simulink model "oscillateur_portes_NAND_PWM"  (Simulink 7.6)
settings: Solver=ode23tb  StartTime=0.0  StopTime=0.01  RelTol=1e-3
InitFcn:
  | clc
StopFcn:
  | close all
  | load es.mat
  | plot(es(1,:),es(2,:))
  | title('Oscillateur PWM à portes NAND')
  | xlabel('temps')
  | grid
  | 
  | delete *.mat
libraries: fl_lib x6, elec_lib x3, nesl_utility x2

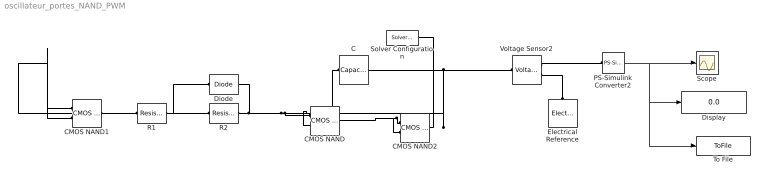
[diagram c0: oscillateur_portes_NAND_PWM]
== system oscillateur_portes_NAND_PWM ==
  C : fl_lib/Electrical/Electrical Elements/Capacitor  DialogController=NetworkEngine.DynNeDlgSource  SystemSampleTime=-1  c=1e-6 F  v0=5 V  r=1e-6 Ohm  g=0 1/Ohm  i_Log=off  v_Log=off  vc_Log=off  LocalVarNames=|i|v|vc  LocalVarDescs=|i|v|Internal variable for voltage across capacitor term  LocalVarLogging=[0 0 0]
  CMOS NAND : elec_lib/Integrated Circuits/Logic/CMOS NAND  DialogController=NetworkEngine.DynNeDlgSource  SystemSampleTime=-1  V_IL=2 V  V_IH=3 V  C_IN=5 pF  output_type=1  V_OL=0 V  V_OH=5 V  V_CC=5 V  V_meas=5 V  R_OUT=25 Ohm  R_OH=[ 25 250 ] Ohm  I_OH=63 mA  R_OL=[ 30 800 ] Ohm  I_OL=-45 mA  Delay=25 ns  Ron=5 Ohm  Vf=0.6 V  output_state=1  LocalVarLogging=[]
  CMOS NAND1 : elec_lib/Integrated Circuits/Logic/CMOS NAND  DialogController=NetworkEngine.DynNeDlgSource  SystemSampleTime=-1  V_IL=2 V  V_IH=3 V  C_IN=5 pF  output_type=1  V_OL=0 V  V_OH=5 V  V_CC=5 V  V_meas=5 V  R_OUT=25 Ohm  R_OH=[ 25 250 ] Ohm  I_OH=63 mA  R_OL=[ 30 800 ] Ohm  I_OL=-45 mA  Delay=25 ns  Ron=5 Ohm  Vf=0.6 V  output_state=1  LocalVarLogging=[]
  CMOS NAND2 : elec_lib/Integrated Circuits/Logic/CMOS NAND  DialogController=NetworkEngine.DynNeDlgSource  SystemSampleTime=-1  V_IL=2 V  V_IH=3 V  C_IN=5 pF  output_type=1  V_OL=0 V  V_OH=5 V  V_CC=5 V  V_meas=5 V  R_OUT=25 Ohm  R_OH=[ 25 250 ] Ohm  I_OH=63 mA  R_OL=[ 30 800 ] Ohm  I_OL=-45 mA  Delay=25 ns  Ron=5 Ohm  Vf=0.6 V  output_state=1  LocalVarLogging=[]
  Diode : fl_lib/Electrical/Electrical Elements/Diode  DialogController=NetworkEngine.DynNeDlgSource  SystemSampleTime=-1  Vf=0.6 V  Ron=0.3 Ohm  Goff=1e-8 1/Ohm  i_Log=off  v_Log=off  LocalVarNames=|i|v  LocalVarDescs=|i|v  LocalVarLogging=[0 0]
  Display : Display
  Electrical Reference : fl_lib/Electrical/Electrical Elements/Electrical Reference  DialogController=NetworkEngine.DynNeDlgSource  SystemSampleTime=-1  i_Log=off  LocalVarNames=|i  LocalVarDescs=|i  LocalVarLogging=0
  PS-Simulink Converter2 : nesl_utility/PS-Simulink Converter  DialogController=NetworkEngine.DynNeUtilDlgSource  SystemSampleTime=-1  PhysicalDomain=network_engine_domain  LeftPortType=input  RightPortType=output  SubClassName=ps_output  Unit=1  AffineConversion=off
  R1 : fl_lib/Electrical/Electrical Elements/Resistor  DialogController=NetworkEngine.DynNeDlgSource  SystemSampleTime=-1  R=0.47 kOhm  i_Log=off  v_Log=off  LocalVarNames=|i|v  LocalVarDescs=|i|v  LocalVarLogging=[0 0]
  R2 : fl_lib/Electrical/Electrical Elements/Resistor  DialogController=NetworkEngine.DynNeDlgSource  SystemSampleTime=-1  R=1.2 kOhm  i_Log=off  v_Log=off  LocalVarNames=|i|v  LocalVarDescs=|i|v  LocalVarLogging=[0 0]
  Scope : Scope
  Solver Configuration : nesl_utility/Solver Configuration  DialogController=NetworkEngine.DynNeUtilDlgSource  SystemSampleTime=-1  PhysicalDomain=network_engine_domain  LeftPortType=input  RightPortType=generic  SubClassName=solver  Accelerate=off  Profile=off  ResidualTolerance=1e-9  MaxNonlinIter=12  MaxModeIter=2  DoFixedCost=off  UseLocalSampling=off  DoDC=off  LinearAlgebra=Sparse  LocalSolverSampleTime=.001  LocalSolverChoice=NE_BACKWARD_EULER_ADVANCER  UseLocalSolver=off
  To File : ToFile  Filename=es.mat  MatrixName=es
  Voltage Sensor2 : fl_lib/Electrical/Electrical Sensors/Voltage Sensor  DialogController=NetworkEngine.DynNeDlgSource  SystemSampleTime=-1  i1_Log=off  v1_Log=off  LocalVarNames=|i1|v1  LocalVarDescs=|i1|v1  LocalVarLogging=[]
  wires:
  PS-Simulink Converter2/1 -> Scope/1, Display/1, To File/1
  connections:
  R2/RConn1 -- CMOS NAND/LConn2 -- CMOS NAND/LConn1 -- C/RConn1 -- Diode/RConn1
  Voltage Sensor2/RConn1 -- PS-Simulink Converter2/LConn1
  Electrical Reference/LConn1 -- Voltage Sensor2/RConn2
  CMOS NAND2/LConn2 -- CMOS NAND2/LConn1 -- CMOS NAND/RConn1
  CMOS NAND1/RConn1 -- R1/LConn1
  CMOS NAND2/RConn1 -- CMOS NAND1/LConn2 -- CMOS NAND1/LConn1 -- Voltage Sensor2/LConn1 -- C/LConn1 -- Solver Configuration/RConn1
  R1/RConn1 -- R2/LConn1 -- Diode/LConn1
